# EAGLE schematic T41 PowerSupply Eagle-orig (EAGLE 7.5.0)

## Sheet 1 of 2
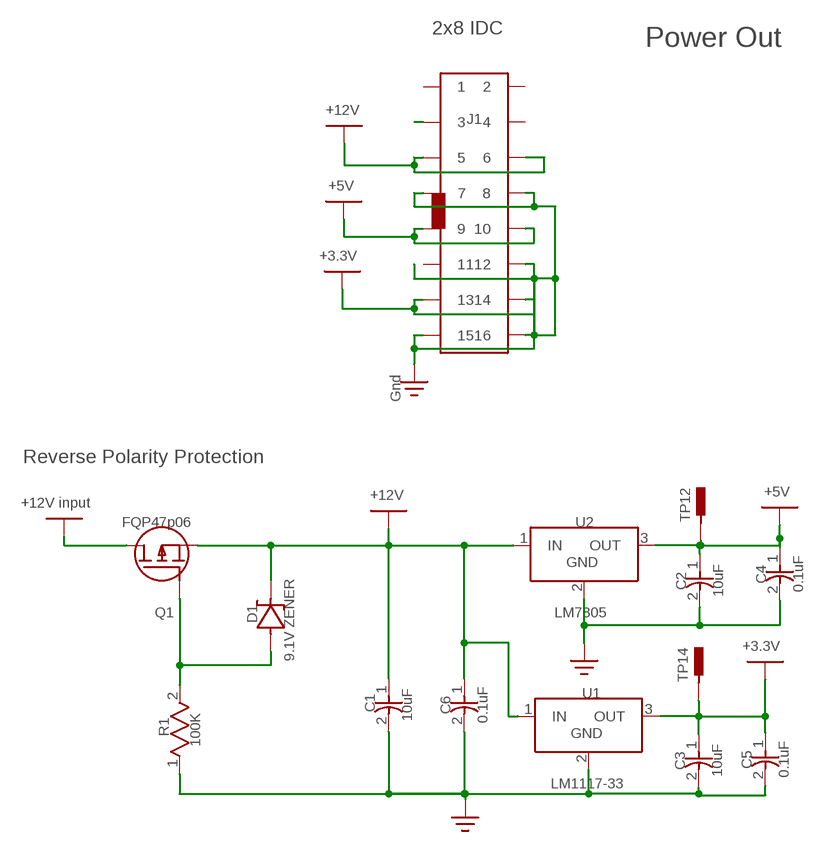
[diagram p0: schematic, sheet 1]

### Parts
C1  10uF  CAP  [CAP-2.54/6.6X3]
C2  10uF  CAP  [CAP-2.54/6.6X3]
C3  10uF  CAP  [CAP-2.54/6.6X3]
C4  0.1uF  CAP  [CAP-2.54/6.6X3]
C5  0.1uF  CAP  [CAP-2.54/6.6X3]
C6  0.1uF  CAP  [CAP-2.54/6.6X3]
D1  9.1V_ZENER  (no package)
J1  2X8IDC  (no package)
Q1  FQP47p06  MOSFET_ENH_P  (no package)
R1  100K  RES_1206  [RES_1206]
TP12  CON_MALE_2  (no package)
TP14  CON_MALE_2  (no package)
U1  LM1117-33  [TO-220]
U2  LM7805  [TO-220]

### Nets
Net_4: J1.7 J1.8 J1.12 J1.15 J1.16 ; supply symbol labelled GND
Net_5: D1.A Q1.G R1.2
Net_6: Q1.D ; supply symbol labelled +12V_INPUT
Net_8: J1.3
Net_132: C1.1 C6.1 D1.K J1.5 J1.6 Q1.S U1.1(IN) U2.1(IN) ; supply symbol labelled +12V
Net_215: C3.1 C5.1 J1.13 J1.14 TP14.1 U1.3(OUT) ; supply symbol labelled +3.3V
Net_222: C2.1 C4.1 J1.9 J1.10 TP12.1 U2.3(OUT) ; supply symbol labelled +5V
Net_234: C1.2 C2.2 C3.2 C4.2 C5.2 C6.2 R1.1 U1.2(GND) U2.2(GND) ; supply symbol labelled MAIN_GND
Unconnected: J1.1 J1.2 J1.4 J1.11

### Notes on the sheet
- 2x8 IDC | Power Out
- +12V
- J1
- +5V
- +3.3V
- Gnd
- Reverse Polarity Protection
- +12V | +5V
- +12V input
- TP12
- FQP47p06 | U2
- GND
- C4
- C2 | 0.1uF
- 10uF
- Q1 | LM7805
- D1
- +3.3V
- 9.1V ZENER
- TP14
- U1
- C1 | C6
- 10uF | 0.1uF
- GND
- R1
- 100K
- C3 | C5
- LM1117-33 | 10uF | 0.1uF

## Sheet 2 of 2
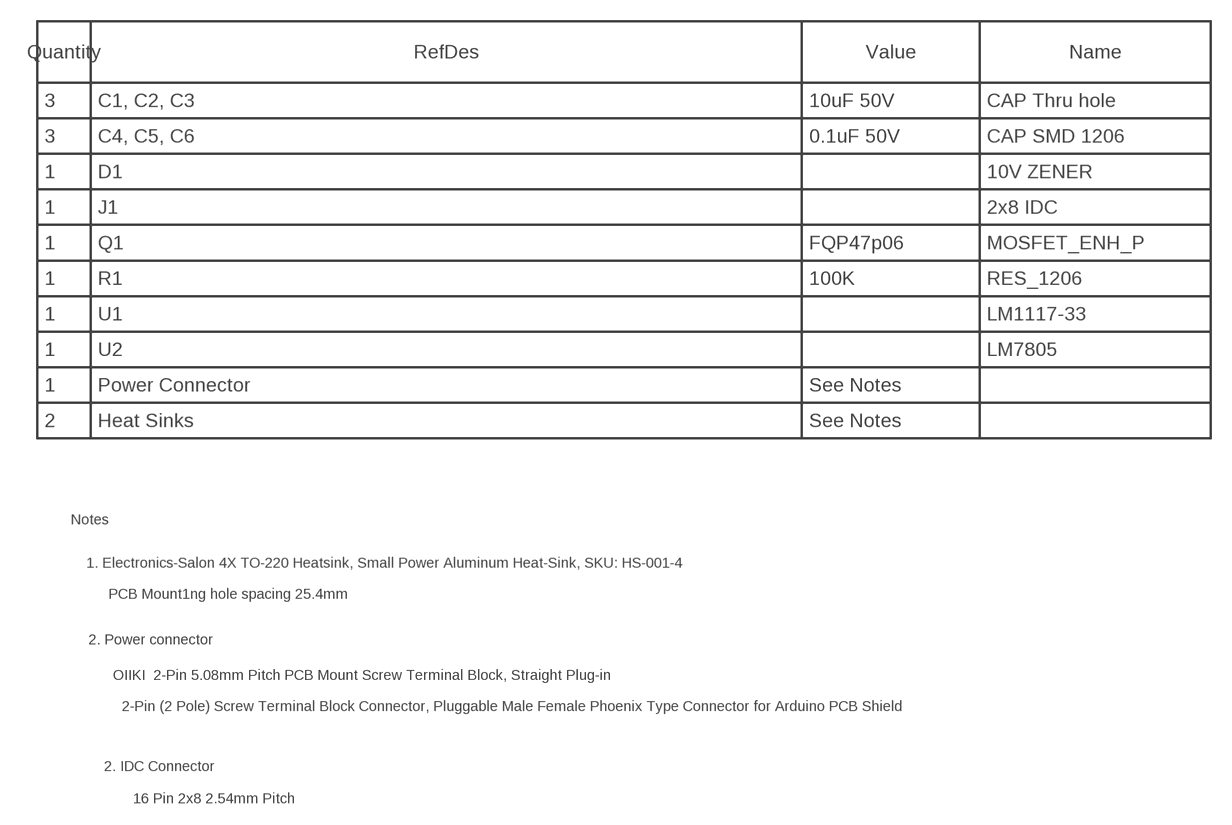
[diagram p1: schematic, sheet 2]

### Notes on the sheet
- Quantity | RefDes | Value | Name
- 3 | C1, C2, C3 | 10uF 50V | CAP Thru hole
- 3 | C4, C5, C6 | 0.1uF 50V | CAP SMD 1206
- 1 | D1 | 10V ZENER
- 1 | J1 | 2x8 IDC
- 1 | Q1 | FQP47p06 | MOSFET_ENH_P
- 1 | R1 | 100K | RES_1206
- 1 | U1 | LM1117-33
- 1 | U2 | LM7805
- 1 | Power Connector | See Notes
- 2 | Heat Sinks | See Notes
- Notes
- 1. Electronics-Salon 4X TO-220 Heatsink, Small Power Aluminum Heat-Sink, SKU: HS-001-4
- PCB Mount1ng hole spacing 25.4mm
- 2. Power connector
- OIIKI  2-Pin 5.08mm Pitch PCB Mount Screw Terminal Block, Straight Plug-in
- 2-Pin (2 Pole) Screw Terminal Block Connector, Pluggable Male Female Phoenix Type Connector for Arduino PCB Shield
- 2. IDC Connector
- 16 Pin 2x8 2.54mm Pitch

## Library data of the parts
C1-C3 = common:CAP
C4-C6 = common:CAP; VALUE: 10uF
D1 = common:9.1V_ZENER; DESCRIPTION: Diode; UNTITLED: Zener
J1 = common:2X8IDC
Q1 = common:MOSFET_ENH_P; DESCRIPTION: MOSFET; UNTITLED: Single-Gate
R1 = common:RES_1206
TP12 TP14 = common:CON_MALE_2; DESCRIPTION: Contact; UNTITLED: Plug
U1 = common:LM1117-33; MANUFACTURER: National Semiconductor
U2 = common:LM7805; MANUFACTURER: National Semiconductor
